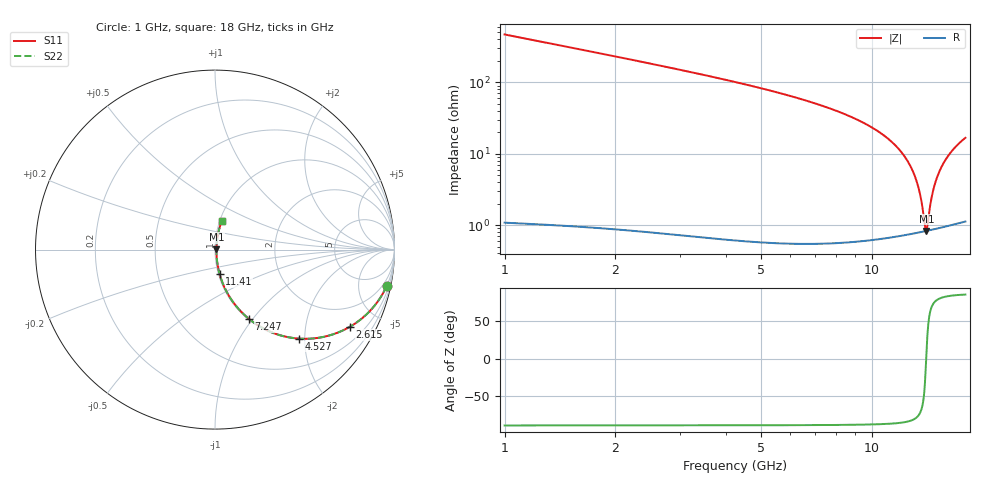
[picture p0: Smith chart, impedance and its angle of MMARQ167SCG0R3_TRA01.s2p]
! MMARQ167SCG0R3_TRA01  S-PARAMETER MODEL  ( General Type )
! Model Generated by TAIYO YUDEN Corporation (http://www.ty-top.com)
! Version 1.0
! TAIYO YUDEN Control No. 180601
! Copyright(c) 2018 TAIYO YUDEN CO.,LTD. All Rights Reserved.
! Product Description (link to TY-COMPAS)
! https://ds.yuden.co.jp/TYCOMPAS/or/detail?pn=MMARQ167SCG0R3ATRA01&u=M
! Products Name : Multilayer Ceramic Capacitors
! Characteristics :
!  Capacitance : 0.3 pF , Rated Voltage : 250V , TCC : CG / C0G
!  Case Size : 1.6 x 0.8 / 0.063 x 0.031 [mm/inch] , Thickness : 0.7 / 0.028 [mm/inch]
!  (Conditions: Temperature = 25 degC , DC Bias Current/Voltage = 0A / 0V)
! External Node Assignments :
!  1  o---| |---o  2
! GND o---------o GND
! Frequency Range : 1000MHz  -  18000MHz  [ 401 STEP ]
# MHz S RI R 50
! Freq[MHz].  S11 Real  S11 Imag  S21 Real  S21 Imag  S12 Real  S12 Imag  S22 Real  S22 Imag
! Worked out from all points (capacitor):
!   401 points, 1 GHz to 18 GHz, reference 50 ohm
!   read as one part in series: C = 337 fF near 1.085 GHz
!   lowest |Z| = 830 mohm at 14.09 GHz (marker M1)
!   series resonance near 14.08 GHz, so ESL is about 380 pH
!   S11 on the Smith chart (normalised r, x): 1 GHz: 1.02, -9.38; 2.615 GHz: 1.02, -3.49; 4.527 GHz: 1.01, -1.87; 7.247 GHz: 1.01, -0.96; 11.41 GHz: 1.01, -0.28; 18 GHz: 1.02, +0.33
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1000  0.9561 -0.2037  0.0439 0.2037  0.0439 0.2037  0.9561 -0.2037
1722.5  0.8784 -0.3251  0.1216 0.3251  0.1216 0.3251  0.8784 -0.3251
2615  0.7515 -0.4299  0.2485 0.4299  0.2485 0.4299  0.7515 -0.4299
3847.5  0.5634 -0.4932  0.4366 0.4932  0.4366 0.4932  0.5634 -0.4932
4527.5  0.4673 -0.4958  0.5327 0.4958  0.5327 0.4958  0.4673 -0.4958
6695  0.2324 -0.4174  0.7676 0.4174  0.7676 0.4174  0.2324 -0.4174
7247.5  0.1898 -0.3865  0.8102 0.3865  0.8102 0.3865  0.1898 -0.3865
9500  0.0733 -0.2498  0.9267 0.2498  0.9267 0.2498  0.0733 -0.2498
11412.5  0.0261 -0.1374  0.9739 0.1374  0.9739 0.1374  0.0261 -0.1374
12347.5  0.0148 -0.0864  0.9852 0.0864  0.9852 0.0864  0.0148 -0.0864
12900  0.0109 -0.0576  0.9891 0.0576  0.9891 0.0576  0.0109 -0.0576
13325  0.00906 -0.0363  0.9909 0.0363  0.9909 0.0363  0.00906 -0.0363
13665  0.00833 -0.0196  0.9917 0.0196  0.9917 0.0196  0.00833 -0.0196
14005  0.00817 -0.00335  0.9918 0.00335  0.9918 0.00335  0.00817 -0.00335
14090  0.00821 0.000653  0.9918 -0.000653  0.9918 -0.000653  0.00821 0.000653
14175  0.00828 0.00463  0.9917 -0.00463  0.9917 -0.00463  0.00828 0.00463
14430  0.0087 0.0164  0.9913 -0.0164  0.9913 -0.0164  0.0087 0.0164
14642.5  0.00925 0.026  0.9907 -0.026  0.9907 -0.026  0.00925 0.026
15195  0.0115 0.0504  0.9885 -0.0504  0.9885 -0.0504  0.0115 0.0504
15705  0.0146 0.072  0.9854 -0.072  0.9854 -0.072  0.0146 0.072
16342.5  0.0195 0.0977  0.9805 -0.0977  0.9805 -0.0977  0.0195 0.0977
18000  0.0373 0.1588  0.9627 -0.1588  0.9627 -0.1588  0.0373 0.1588
